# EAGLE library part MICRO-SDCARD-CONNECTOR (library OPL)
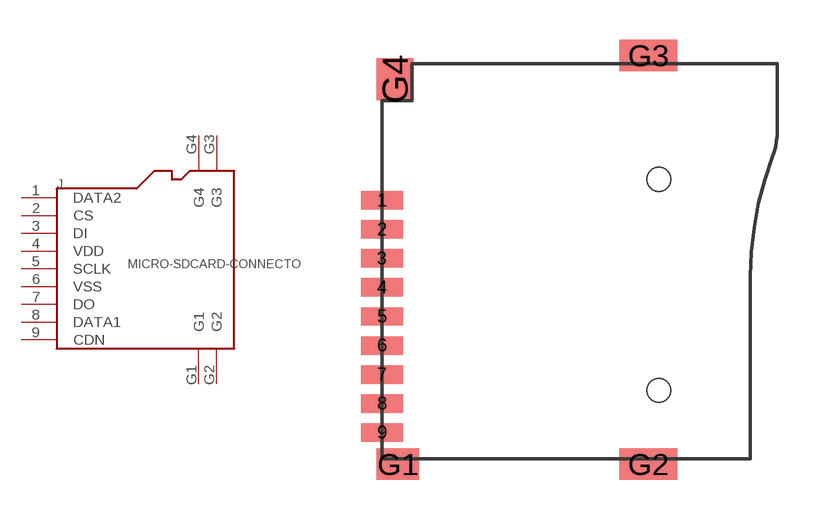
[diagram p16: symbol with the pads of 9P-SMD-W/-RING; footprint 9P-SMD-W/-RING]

Designator prefix J

## MICRO-SDCARD-CONNECTOR-3300060P1  [9P-SMD-W/-RING]
1  DATA2
2  CS
3  DI
4  VDD
5  SCLK
6  VSS
7  DO
8  DATA1
9  CDN
G1  G1
G2  G2
G3  G3
G4  G4

## Footprint 9P-SMD-W/-RING (pad centres in mm)
smd 1.6 x 0.7: 1 0,2.25; 2 0,1.15; 3 0,0.05; 4 0,-1.05; 5 0,-2.15; 6 0,-3.25; 7 0,-4.35; 8 0,-5.45; 9 0,-6.55
smd 1.6 x 1.2: G1 0.6,-7.75
smd 2.2 x 1.2: G2 10.1,-7.75; G3 10.1,7.75
smd 1.4 x 1.6: G4 0.5,6.85
hole 0.9 at 10.5,-4.95
hole 0.9 at 10.5,3.05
